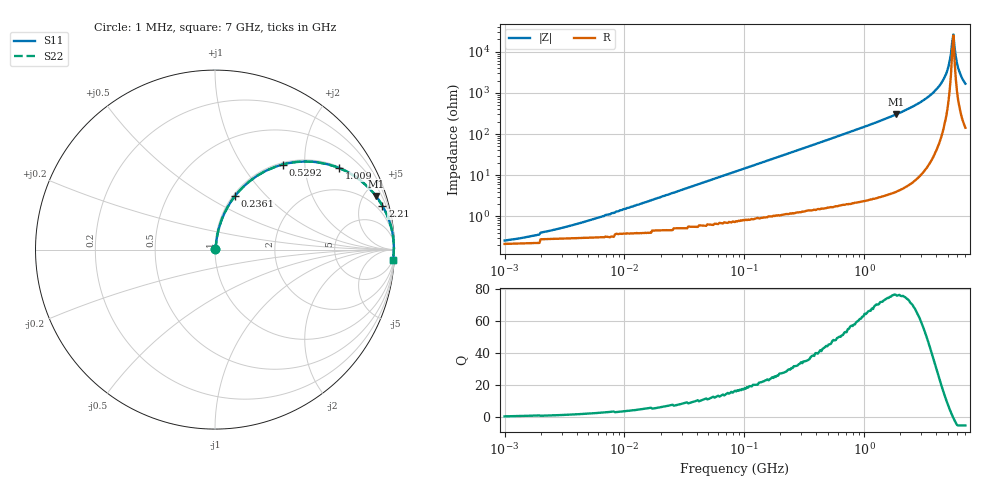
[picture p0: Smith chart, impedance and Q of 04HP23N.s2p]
# MHz S MA R 50
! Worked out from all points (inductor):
!   385 points, 1 MHz to 7 GHz, reference 50 ohm
!   read as one part in series: L = 23 nH near 6.473 MHz
!   highest Q = 76.4 at 1.838 GHz (marker M1), where L = 25.9 nH
!   self-resonance near 5.432 GHz
!   S11 on the Smith chart (normalised r, x): 1 MHz: 1.00, +0.00; 236.1 MHz: 1.02, +0.68; 529.2 MHz: 1.03, +1.54; 1.009 GHz: 1.05, +3.02; 2.21 GHz: 1.10, +7.60; 7 GHz: 4, -33
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1  0.002661 32.7  0.998 -0.1  0.998 -0.1  0.002661 32.7
4.374  0.006951 64.7  0.997 -0.4  0.997 -0.4  0.006951 64.7
19.575  0.028 79.5  0.995 -1.6  0.995 -1.6  0.028 79.5
85.617  0.122 79.5  0.985 -7.0  0.985 -7.0  0.122 79.5
236.127  0.32 69.4  0.937 -18.7  0.937 -18.7  0.32 69.4
365.931  0.464 60.8  0.874 -27.6  0.874 -27.6  0.464 60.8
529.189  0.605 51.6  0.783 -37.2  0.783 -37.2  0.605 51.6
1009.213  0.828 33.3  0.549 -55.8  0.549 -55.8  0.828 33.3
1637.803  0.929 21.0  0.358 -68.3  0.358 -68.3  0.929 21.0
1837.926  0.945 18.4  0.316 -70.8  0.316 -70.8  0.945 18.4
2210.214  0.964 14.7  0.254 -74.5  0.254 -74.5  0.964 14.7
3347.135  0.989 7.4  0.13 -81.4  0.13 -81.4  0.989 7.4
4414.002  0.996 3.2  0.057 -83.9  0.057 -83.9  0.996 3.2
4840.449  0.996 1.9  0.034 -82.8  0.034 -82.8  0.996 1.9
5068.882  0.997 1.3  0.022 -80.4  0.022 -80.4  0.997 1.3
5308.095  0.997 0.6  0.011 -71.3  0.011 -71.3  0.997 0.6
5431.903  0.997 0.3  0.005734 -52.5  0.005734 -52.5  0.997 0.3
5558.598  0.996 -0.1  0.003763 18.2  0.003763 18.2  0.996 -0.1
5688.248  0.996 -0.4  0.007842 61.6  0.007842 61.6  0.996 -0.4
5956.691  0.996 -1.1  0.019 76.9  0.019 76.9  0.996 -1.1
6383.295  0.995 -2.0  0.036 81.0  0.036 81.0  0.995 -2.0
7000  0.993 -3.4  0.059 81.8  0.059 81.8  0.993 -3.4
